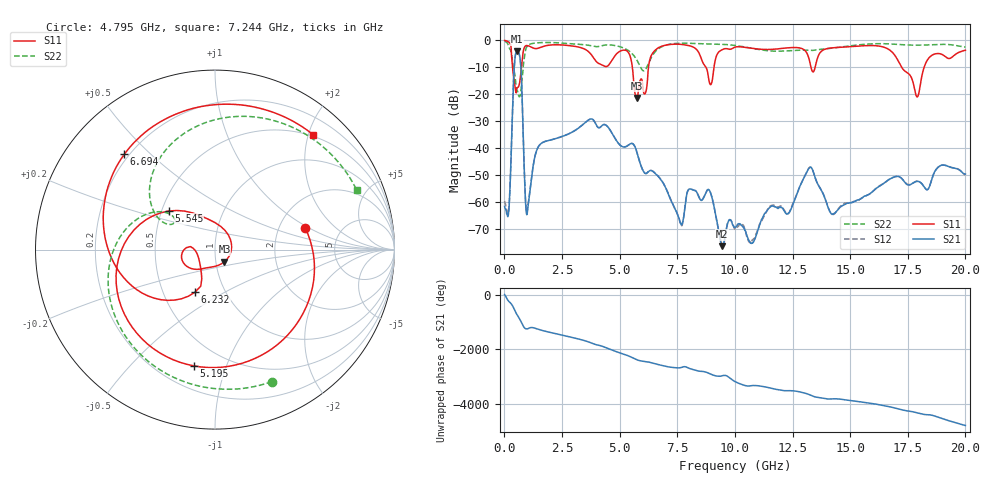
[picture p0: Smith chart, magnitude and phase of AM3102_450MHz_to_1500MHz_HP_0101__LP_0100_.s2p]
!Agilent Technologies,E8364B,MY43040894,A.07.50.67
!Agilent E8364B: A.07.50.67
!Date: Thursday, January 11, 2018 05:40:46
!Correction: S11(Full 2 Port(1,2))
!S21(Full 2 Port(1,2))
!S12(Full 2 Port(1,2))
!S22(Full 2 Port(1,2))
!S2P File: Measurements: S11, S21, S12, S22:
# Hz S  dB  R 50
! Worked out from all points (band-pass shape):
!   1601 points, 10 MHz to 20 GHz, reference 50 ohm
!   highest |S21| = -4.05 dB at 559.7 MHz (marker M1); lowest = -76.3 dB at 9.455 GHz (marker M2)
!   |S21| within 3 dB of the highest: 455.7 MHz to 686.1 MHz (230.4 MHz wide, 40.4 % of centre)
!   lowest |S11| = -21.3 dB at 5.745 GHz (marker M3), VSWR 1.19, Z = 55 - j7.51 ohm
!   |S11| at or under -10 dB: 353.2 MHz to 739.9 MHz (386.6 MHz wide, 70.7 % of centre); 5.552 GHz to 6.252 GHz (699.1 MHz wide, 11.8 % of centre); 17.24 GHz to 18.21 GHz (973.4 MHz wide, 5.49 % of centre)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
!   |S22| runs from -20.9 to -0.3 dB; largest |S21 - S12| = 0.0014
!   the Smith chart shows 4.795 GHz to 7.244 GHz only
!   S11 on the Smith chart (normalised r, x): 4.795 GHz: 2.81, +0.91; 5.195 GHz: 0.34, -0.78; 5.545 GHz: 0.55, +0.26; 6.232 GHz: 0.72, -0.37; 6.694 GHz: 0.18, +0.42; 7.244 GHz: 0.48, +2.09
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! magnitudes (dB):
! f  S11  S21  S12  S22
! 10 MHz  -0.1  -61.5  -59.5  -0.3
! 197.4 MHz  -0.7  -62.4  -62.0  -2.5
! 559.7 MHz  -17.6  -4.0  -4.0  -18.7
! 997 MHz  -2.0  -63.7  -63.0  -2.1
! 1.509 GHz  -2.8  -39.0  -39.0  -0.9
! 3.346 GHz  -2.8  -31.6  -31.6  -1.5
! 4.795 GHz  -5.7  -36.2  -36.2  -1.9
! 5.195 GHz  -3.6  -39.5  -39.5  -2.9
! 5.545 GHz  -9.5  -38.2  -38.2  -5.0
! 5.745 GHz  -21.3  -41.3  -41.4  -7.3
! 6.232 GHz  -11.6  -48.8  -48.7  -8.9
! 6.682 GHz  -2.8  -50.5  -50.4  -3.1
! 6.694 GHz  -2.7  -50.6  -50.5  -3.1
! 7.244 GHz  -1.5  -59.7  -59.5  -1.3
! 8.881 GHz  -15.1  -55.4  -55.4  -1.3
! 9.455 GHz  -3.5  -76.3  -76.1  -1.5
! 10.01 GHz  -2.5  -69.3  -69.8  -1.9
! 13.34 GHz  -11.2  -47.5  -47.5  -3.8
! 14.25 GHz  -2.8  -64.4  -64.4  -2.9
! 16.68 GHz  -3.4  -51.6  -51.6  -1.3
! 17.9 GHz  -21.0  -52.3  -52.1  -1.8
! 20 GHz  -3.7  -49.5  -49.9  -2.5
